TYPE "KOM Sw->Ext"
TITLE =Kommunikationssignale nach Extern
AUTHOR : dfb
FAMILY : KOM
NAME : 'SwAP&T'
VERSION : 0.1


  STRUCT
OUT: STRUCT //Ausgangssignale
LifeBit : Bool ;  //Life bit communication
EmStopOK : Bool ;  //Emergency stop furnace OK
NoWarning : Bool ;  //No warning furnace
NoError : Bool ;  //No error furnace
Spare_0_4 : Bool ;  //Reserve
Spare_0_5 : Bool ;  //Reserve
Spare_0_6 : Bool ;  //Reserve
Spare_0_7 : Bool ;  //Reserve
StopCycleEndZ1 : Bool ;  //Stop at cycle end reached zone press cell (OK open guards)
StopCycleEndZ2 : Bool ;  //Stop at cycle end reached zone loading furnace (OK open guards)
Auto_Selected : Bool ;  //OP mode Auto selected
Auto_Active : Bool ;  //Auto mode furnace active (machine is running in continous)
OKChangeRecipe : Bool ;  //OK to change recipe in Furnace
Spare_1_5 : Bool ;  //Reserve
Spare_1_6 : Bool ;  //Reserve
Rob2_OkToLeave : Bool ;  //OK leave parts loading zone
Part_OnTheWay : Bool ;  //Parts on the way
Part1_InPos : Bool ;  //Part 1 in position
Part2_InPos : Bool ;  //Part 2 in position
Part3_InPos : Bool ;  //Part 3 in position
Part4_InPos : Bool ;  //Part 4 in position
PartsCentered : Bool ;  //Parts centered on furnace
PartsOKHeatT : Bool ;  //Parts OK heat treated
PartsNotOKHeatT : Bool ;  //Parts not OK heat treated
Spare_3_0 : Bool ;  //Reserve
Spare_3_1 : Bool ;  //Reserve
Spare_3_2 : Bool ;  //Reserve
Spare_3_3 : Bool ;  //Reserve
Spare_3_4 : Bool ;  //Reserve
Spare_3_5 : Bool ;  //Reserve
Spare_3_6 : Bool ;  //Reserve
Spare_3_7 : Bool ;  //Reserve
Spare_4_0 : Bool ;  //Furnace in stop , status signal (Special for Fiat)
Spare_4_1 : Bool ;  //Furnace ready , status signal (Special for Fiat)
Spare_4_2 : Bool ;  //Furnace standby , status signal (Special for Fiat)
Spare_4_3 : Bool ;  //Furnace producing, status signal (Special for Fiat)
Spare_4_4 : Bool ;  //Furnace manual mode, status signal (Special for Fiat)
Spare_4_5 : Bool ;  //Furnace alarm, status signal (Special for Fiat)
Spare_4_6 : Bool ;  //Reserve
Spare_4_7 : Bool ;  //Reserve
Spare_5_0 : Bool ;  //Reserve
Spare_5_1 : Bool ;  //Reserve
Spare_5_2 : Bool ;  //Reserve
Spare_5_3 : Bool ;  //Reserve
Spare_5_4 : Bool ;  //Reserve
Spare_5_5 : Bool ;  //Reserve
Spare_5_6 : Bool ;  //Reserve
Spare_5_7 : Bool ;  //Reserve
ActiveRecipeNo : INT ;  //Activce recipe number in furnace
Spare_8_0 : INT ;  //Reserve
END_STRUCT ;
END_STRUCT ;
END_TYPE
